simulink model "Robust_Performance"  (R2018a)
settings: Solver=ode113  StartTime=0.0  StopTime=20  FixedStep=0.0001  RelTol=1e-5  EnableMultiTasking=on
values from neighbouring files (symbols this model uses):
  d2r = pi/180    (= 0.0174532925199)    [init.m]
  Kr = Kq; Kr(3:4)=-Kq(3:4)    [init.m]
  Npv = 19    [init.m]    (also in Run_Robust_Performance.m; Run_Robustness.m)
  r2d = 1/d2r    (= 57.2957795131)    [init.m]
  Wf = 20    [init.m]
undefined symbols (not defined in the file or in its folder): Aa, Av, Ba, Bv, Ca, Cv, Da, Dv, Kq, TVC

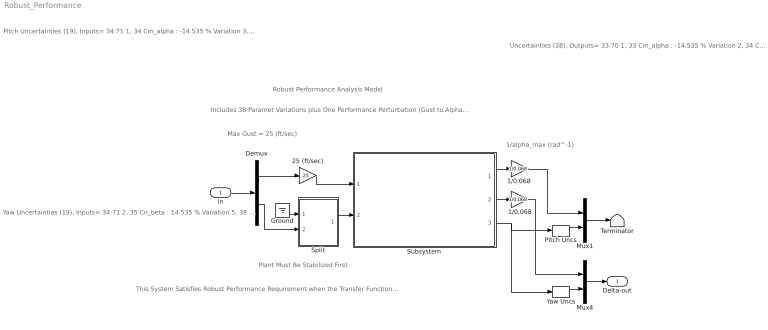
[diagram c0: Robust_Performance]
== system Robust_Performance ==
  note: Robust Performance Analysis Model
  note: Uncertainties (38), Outputs= 33:70 1, 33 Cm_alpha : -14.535 % Variation 2, 34 Cn_beta : 14.535 % Variation 3, 35 Ca_alpha : 17.153 % Variation 4, 36 Cz_alpha : -24.655 % Variation 5, 37 Cy_beta : -24.655 % Variation 6, 38 Cm_0 : -9.690 % Variation 7, 39 CZ_0 : -12.327 % Variation 8, 40 CA_0 : 6.679 % Variation 9, 41 I_xx : 19.786 % Variation 10, 42 I_yy : 14.153 % Variation 11, 43 I_zz : 14.158 % Variation 12, 44 Qbar : 9.865 % Variation 13, 45 Qbar : 9.865 % Variation 14, 46 Xcg locat: 3.492 % Variation 15, 47 Xcg locat: 3.492 % Variation 16, 48 Xcg locat: 3.492 % Variation 17, 49 M_slosh 1: 13.664 % Variation 18, 50 M_slosh 1: 13.664 % Variation 19, 51 X_slosh 1: 3.563 % Variation 20, 52 X_slosh 1: 3.563 % Variation 21, 53 X_slosh 1: 3.563 % Variation 22, 54 Wslsh_Y 1: 2.251 % Variation 23, 55 Wslsh_Z 1: 2.251 % Variation 24, 56 ZetSl_Y 1: 5.556 % Variation 25, 57 ZetSl_Z 1: 5.556 % Variation 26, 58 M_slosh 2: 14.465 % Variation 27, 59 M_slosh 2: 14.465 % Variation 28, 60 X_slosh 2: 7.956 % Variation 29, 61 X_slosh 2: 7.956 % Variation 30, 62 X_slosh 2: 7.956 % Variation 31, 63 Wslsh_Y 2: 2.251 % Variation 32, 64 Wslsh_Z 2: 2.251 % Variation 33, 65 ZetSl_Y 2: 6.667 % Variation 34, 66 ZetSl_Z 2: 6.667 % Variation 35, 67 W_flex 1: 5.000 Addit. Variat. 36, 68 W_flex 2: 5.000 Addit. Variat. 37, 69 W_flex 3: 8.000 Addit. Variat. 38, 70 W_flex 4: 8.000 Addit. Variat.
  note: Plant Must Be Stabilized First
  note: Includes 38 Paramet Variations plus One Performance Perturbation (Gust to Alpha or Beta)
  note: Pitch Uncertainties (19), Inputs= 34:71 1, 34 Cm_alpha : -14.535 % Variation 3, 36 Ca_alpha : 17.153 % Variation 4, 37 Cz_alpha : -24.655 % Variation 6, 39 Cm_0 : -9.690 % Variation 7, 40 CZ_0 : -12.327 % Variation 8, 41 CA_0 : 6.679 % Variation 10, 43 I_yy : 14.153 % Variation 12, 45 Qbar : 9.865 % Variation 15, 48 Xcg locat: 3.492 % Variation 18, 51 M_slosh 1: 13.664 % Variation 20, 53 X_slosh 1: 3.563 % Variation 23, 56 Wslsh_Z 1: 2.251 % Variation 25, 58 ZetSl_Z 1: 5.556 % Variation 27, 60 M_slosh 2: 14.465 % Variation 29, 62 X_slosh 2: 7.956 % Variation 32, 65 Wslsh_Z 2: 2.251 % Variation 34, 67 ZetSl_Z 2: 6.667 % Variation 36, 69 W_flex 2: 5.000 Addit. Variat. 38, 71 W_flex 4: 8.000 Addit. Variat.
  note: Yaw Uncertainties (19), Inputs= 34:71 2, 35 Cn_beta : 14.535 % Variation 5, 38 Cy_beta : -24.655 % Variation 9, 42 I_xx : 19.786 % Variation 11, 44 I_zz : 14.158 % Variation 13, 46 Qbar : 9.865 % Variation 14, 47 Xcg locat: 3.492 % Variation 16, 49 Xcg locat: 3.492 % Variation 17, 50 M_slosh 1: 13.664 % Variation 19, 52 X_slosh 1: 3.563 % Variation 21, 54 X_slosh 1: 3.563 % Variation 22, 55 Wslsh_Y 1: 2.251 % Variation 24, 57 ZetSl_Y 1: 5.556 % Variation 26, 59 M_slosh 2: 14.465 % Variation 28, 61 X_slosh 2: 7.956 % Variation 30, 63 X_slosh 2: 7.956 % Variation 31, 64 Wslsh_Y 2: 2.251 % Variation 33, 66 ZetSl_Y 2: 6.667 % Variation 35, 68 W_flex 1: 5.000 Addit. Variat. 37, 70 W_flex 3: 8.000 Addit. Variat.
  note: 1/alpha_max (rad^-1)
  note: Max Gust = 25 (ft/sec)
  note: This System Satisfies Robust Performance Requirement when the Transfer Function Magnitude is Less than One at All Frequencies. It Means that it will satisfy Both Performance to Gusts and its Stability will be Robust to All Parameter Variations Defined
  In : Inport
  1/0.068 : Gain  Gain=1/0.068
  "1/0.068 " : Gain  Gain=1/0.068
  25 (ft/sec) : Gain  Gain=25
  Demux : Demux  Outputs=[1, Npv]
  Ground : Ground
  Mux1 : Mux  Inputs=[1, Npv]
  Mux4 : Mux  Inputs=[1, Npv]
  Pitch Uncs : Selector  InputPortWidth=38  IndexOptions=Index vector (dialog)  Indices=[1,3,4,6,7,8,10,12,15,18,20,23,25,27,29,32,34,36,38]  OutputSizes=1
  Split : Subsystem
  Subsystem : Subsystem
  Terminator : Terminator
  Yaw Uncs : Selector  InputPortWidth=38  IndexOptions=Index vector (dialog)  Indices=[2,5,9,11,13,14,16,17,19,21,22,24,26,28,30,31,33,35,37]  OutputSizes=1
  Delta-out : Outport
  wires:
  Split/1(Delta-In) -> Subsystem/2(del-in)
  Subsystem/3(del-out) -> Yaw Uncs/1, Pitch Uncs/1
  Subsystem/2("beta ") -> 1/0.068/1
  Yaw Uncs/1 -> Mux4/2
  Subsystem/1(alpha) -> "1/0.068 "/1
  Pitch Uncs/1 -> Mux1/2
  In/1 -> Demux/1
  Demux/1 -> 25 (ft/sec)/1
  25 (ft/sec)/1 -> Subsystem/1(gust)
  "1/0.068 "/1 -> Mux1/1
  1/0.068/1 -> Mux4/1
  Ground/1 -> Split/1(Pitch)
  Demux/2 -> Split/2(Yaw)
  Mux4/1 -> Delta-out/1
  Mux1/1 -> Terminator/1

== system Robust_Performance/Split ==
  note: Pitch Uncertainties (19), Inputs= 34:71 1, 34 Cm_alpha : -14.535 % Variation 3, 36 Ca_alpha : 17.153 % Variation 4, 37 Cz_alpha : -24.655 % Variation 6, 39 Cm_0 : -9.690 % Variation 7, 40 CZ_0 : -12.327 % Variation 8, 41 CA_0 : 6.679 % Variation 10, 43 I_yy : 14.153 % Variation 12, 45 Qbar : 9.865 % Variation 15, 48 Xcg locat: 3.492 % Variation 18, 51 M_slosh 1: 13.664 % Variation 20, 53 X_slosh 1: 3.563 % Variation 23, 56 Wslsh_Z 1: 2.251 % Variation 25, 58 ZetSl_Z 1: 5.556 % Variation 27, 60 M_slosh 2: 14.465 % Variation 29, 62 X_slosh 2: 7.956 % Variation 32, 65 Wslsh_Z 2: 2.251 % Variation 34, 67 ZetSl_Z 2: 6.667 % Variation 36, 69 W_flex 2: 5.000 Addit. Variat. 38, 71 W_flex 4: 8.000 Addit. Variat.
  note: Uncertainties (38), Inputs= 34:71 1, 34 Cm_alpha : -14.535 % Variation 2, 35 Cn_beta : 14.535 % Variation 3, 36 Ca_alpha : 17.153 % Variation 4, 37 Cz_alpha : -24.655 % Variation 5, 38 Cy_beta : -24.655 % Variation 6, 39 Cm_0 : -9.690 % Variation 7, 40 CZ_0 : -12.327 % Variation 8, 41 CA_0 : 6.679 % Variation 9, 42 I_xx : 19.786 % Variation 10, 43 I_yy : 14.153 % Variation 11, 44 I_zz : 14.158 % Variation 12, 45 Qbar : 9.865 % Variation 13, 46 Qbar : 9.865 % Variation 14, 47 Xcg locat: 3.492 % Variation 15, 48 Xcg locat: 3.492 % Variation 16, 49 Xcg locat: 3.492 % Variation 17, 50 M_slosh 1: 13.664 % Variation 18, 51 M_slosh 1: 13.664 % Variation 19, 52 X_slosh 1: 3.563 % Variation 20, 53 X_slosh 1: 3.563 % Variation 21, 54 X_slosh 1: 3.563 % Variation 22, 55 Wslsh_Y 1: 2.251 % Variation 23, 56 Wslsh_Z 1: 2.251 % Variation 24, 57 ZetSl_Y 1: 5.556 % Variation 25, 58 ZetSl_Z 1: 5.556 % Variation 26, 59 M_slosh 2: 14.465 % Variation 27, 60 M_slosh 2: 14.465 % Variation 28, 61 X_slosh 2: 7.956 % Variation 29, 62 X_slosh 2: 7.956 % Variation 30, 63 X_slosh 2: 7.956 % Variation 31, 64 Wslsh_Y 2: 2.251 % Variation 32, 65 Wslsh_Z 2: 2.251 % Variation 33, 66 ZetSl_Y 2: 6.667 % Variation 34, 67 ZetSl_Z 2: 6.667 % Variation 35, 68 W_flex 1: 5.000 Addit. Variat. 36, 69 W_flex 2: 5.000 Addit. Variat. 37, 70 W_flex 3: 8.000 Addit. Variat. 38, 71 W_flex 4: 8.000 Addit. Variat.
  note: Yaw Uncertainties (19), Inputs= 34:71 2, 35 Cn_beta : 14.535 % Variation 5, 38 Cy_beta : -24.655 % Variation 9, 42 I_xx : 19.786 % Variation 11, 44 I_zz : 14.158 % Variation 13, 46 Qbar : 9.865 % Variation 14, 47 Xcg locat: 3.492 % Variation 16, 49 Xcg locat: 3.492 % Variation 17, 50 M_slosh 1: 13.664 % Variation 19, 52 X_slosh 1: 3.563 % Variation 21, 54 X_slosh 1: 3.563 % Variation 22, 55 Wslsh_Y 1: 2.251 % Variation 24, 57 ZetSl_Y 1: 5.556 % Variation 26, 59 M_slosh 2: 14.465 % Variation 28, 61 X_slosh 2: 7.956 % Variation 30, 63 X_slosh 2: 7.956 % Variation 31, 64 Wslsh_Y 2: 2.251 % Variation 33, 66 ZetSl_Y 2: 6.667 % Variation 35, 68 W_flex 1: 5.000 Addit. Variat. 37, 70 W_flex 3: 8.000 Addit. Variat.
  Pitch : Inport
  Yaw : Inport  Port=2
  Demux : Demux  Outputs=19
  Demux1 : Demux  Outputs=19
  Mux : Mux  Inputs=38
  Delta-In : Outport
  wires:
  Pitch/1 -> Demux/1
  Demux/1 -> Mux/1
  Demux/2 -> Mux/3
  Demux/4 -> Mux/6
  Demux/3 -> Mux/4
  Demux/5 -> Mux/7
  Demux/6 -> Mux/8
  Demux/7 -> Mux/10
  Demux/8 -> Mux/12
  Demux/9 -> Mux/15
  Demux/10 -> Mux/18
  Demux/11 -> Mux/20
  Demux/12 -> Mux/23
  Demux/13 -> Mux/25
  Demux/14 -> Mux/27
  Demux/15 -> Mux/29
  Demux/16 -> Mux/32
  Demux/17 -> Mux/34
  Demux/18 -> Mux/36
  Demux/19 -> Mux/38
  Yaw/1 -> Demux1/1
  Demux1/19 -> Mux/37
  Demux1/18 -> Mux/35
  Demux1/17 -> Mux/33
  Demux1/16 -> Mux/31
  Demux1/15 -> Mux/30
  Demux1/14 -> Mux/28
  Demux1/13 -> Mux/26
  Demux1/12 -> Mux/24
  Demux1/11 -> Mux/22
  Demux1/10 -> Mux/21
  Demux1/9 -> Mux/19
  Demux1/8 -> Mux/17
  Demux1/7 -> Mux/16
  Demux1/1 -> Mux/2
  Demux1/2 -> Mux/5
  Demux1/3 -> Mux/9
  Demux1/4 -> Mux/11
  Demux1/5 -> Mux/13
  Demux1/6 -> Mux/14
  Mux/1 -> Delta-In/1

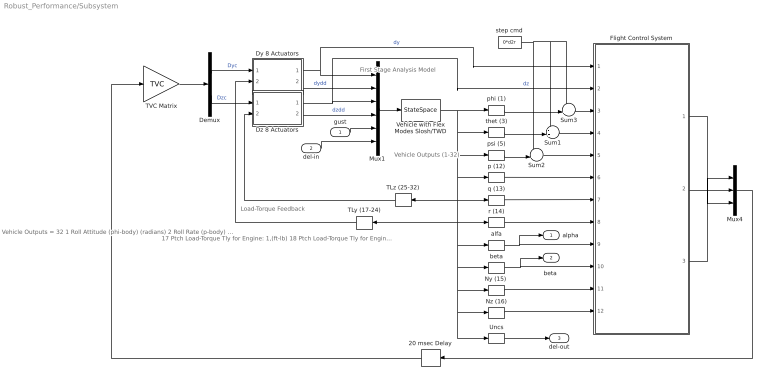
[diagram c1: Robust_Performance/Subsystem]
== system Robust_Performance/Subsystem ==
  note: First Stage Analysis Model
  note: Load-Torque Feedback
  note: 17 Ptch Load-Torque Tly for Engine: 1,(ft-lb) 18 Ptch Load-Torque Tly for Engine: 2,(ft-lb) 19 Ptch Load-Torque Tly for Engine: 3,(ft-lb) 20 Ptch Load-Torque Tly for Engine: 4,(ft-lb) 21 Ptch Load-Torque Tly for Engine: 5,(ft-lb) 22 Ptch Load-Torque Tly for Engine: 6,(ft-lb) 23 Ptch Load-Torque Tly for Engine: 7,(ft-lb) 24 Ptch Load-Torque Tly for Engine: 8,(ft-lb) 25 Yaw Load-Torque Tlz for Engine: 1,(ft-lb) 26 Yaw Load-Torque Tlz for Engine: 2,(ft-lb) 27 Yaw Load-Torque Tlz for Engine: 3,(ft-lb) 28 Yaw Load-Torque Tlz for Engine: 4,(ft-lb) 29 Yaw Load-Torque Tlz for Engine: 5,(ft-lb) 30 Yaw Load-Torque Tlz for Engine: 6,(ft-lb) 31 Yaw Load-Torque Tlz for Engine: 7,(ft-lb) 32 Yaw Load-Torque Tlz for Engine: 8,(ft-lb)
  note: Vehicle Outputs = 32 1 Roll Attitude (phi-body) (radians) 2 Roll Rate (p-body) (rad/sec) 3 Pitch Attitude (thet-bdy) (radians) 4 Pitch Rate (q-body) (rad/sec) 5 Yaw Attitude (psi-body) (radians) 6 Yaw Rate (r-body) (rad/sec) 7 Angle of attack, alfa, (radians) 8 Angle of sideslip, beta, (radian) 9 Change in Altitude, delta-h, (feet) 10 Forward Acceleration (V-dot) (ft/sec) 11 Cross Range Velocity (Vcr) (ft/sec) 12 Rate-Gyro # 1, Roll Rate (Body) (rad/sec) 13 Rate-Gyro # 2, Pitch Rate (Body) (rad/sec) 14 Rate-Gyro # 3, Yaw Rate (Body) (rad/sec) 15 Accelerom # 1, (along Y), (ft/sec^2) Translat. Accelerat. 16 Accelerom # 2, (along Z), (ft/sec^2) Translat. Accelerat.
  note: Vehicle Outputs (1-32)
  gust : Inport
  del-in : Inport  Port=2
  20 msec Delay : TransportDelay  DelayTime="[1  1  1]*0.02"  InitialOutput="[0  0  0]"  PadeOrder=2
  Demux : Demux  Outputs=[8, 8]
  Dy 8 Actuators : Subsystem
  Dz 8 Actuators : Subsystem
  Flight Control System : Subsystem
  Mux1 : Mux  Inputs=[8, 8, 8, 8, 1, 38]
  Mux4 : Mux  Inputs=3
  "Ny (15) " : Selector  InputPortWidth=70  IndexOptions=Index vector (dialog)  Indices=[15]  OutputSizes=1
  Nz (16) : Selector  InputPortWidth=70  IndexOptions=Index vector (dialog)  Indices=[16]  OutputSizes=1
  Sum1 : Sum  Inputs=-+|
  Sum2 : Sum  Inputs=-+|
  Sum3 : Sum  Inputs=-+|
  TLy (17-24) : Selector  InputPortWidth=70  IndexOptions=Index vector (dialog)  Indices=[17:24]  OutputSizes=1
  TLz (25-32) : Selector  InputPortWidth=70  IndexOptions=Index vector (dialog)  Indices=[25:32]  OutputSizes=1
  TVC Matrix : Gain  Gain=TVC  Multiplication=Matrix(K*u)
  Uncs : Selector  InputPortWidth=70  IndexOptions=Index vector (dialog)  Indices=[33:70]  OutputSizes=1
  Vehicle with Flex Modes Slosh/TWD : StateSpace  A=Av  B=Bv  C=Cv  D=Dv  InitialCondition=0
  alfa : Selector  InputPortWidth=70  IndexOptions=Index vector (dialog)  Indices=[7]  OutputSizes=1
  beta : Selector  InputPortWidth=70  IndexOptions=Index vector (dialog)  Indices=[8]  OutputSizes=1
  p (12) : Selector  InputPortWidth=70  IndexOptions=Index vector (dialog)  Indices=[12]  OutputSizes=1
  phi (1) : Selector  InputPortWidth=70  IndexOptions=Index vector (dialog)  Indices=[1]  OutputSizes=1
  psi (5) : Selector  InputPortWidth=70  IndexOptions=Index vector (dialog)  Indices=[5]  OutputSizes=1
  q (13) : Selector  InputPortWidth=70  IndexOptions=Index vector (dialog)  Indices=[13]  OutputSizes=1
  r (14) : Selector  InputPortWidth=70  IndexOptions=Index vector (dialog)  Indices=[14]  OutputSizes=1
  step cmd : Constant  Value=0*d2r
  thet (3) : Selector  InputPortWidth=70  IndexOptions=Index vector (dialog)  Indices=[3]  OutputSizes=1
  alpha : Outport
  "beta " : Outport  Port=2
  del-out : Outport  Port=3
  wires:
  Mux1/1 -> Vehicle with Flex Modes Slosh/TWD/1
  Dz 8 Actuators/2(dzdd) -> Mux1/4  "dzdd"
  p (12)/1 -> Flight Control System/6(p)
  Vehicle with Flex Modes Slosh/TWD/1 -> TLz (25-32)/1, "Ny (15) "/1, Uncs/1, Nz (16)/1, beta/1, alfa/1, TLy (17-24)/1, r (14)/1, q (13)/1, p (12)/1, psi (5)/1, thet (3)/1, phi (1)/1
  20 msec Delay/1 -> TVC Matrix/1
  TVC Matrix/1 -> Demux/1
  gust/1 -> Mux1/5
  del-in/1 -> Mux1/6
  "Ny (15) "/1 -> Flight Control System/11(NY)
  Dz 8 Actuators/1(dz) -> Flight Control System/2(dz), Mux1/3  "dz"
  r (14)/1 -> Flight Control System/8(r)
  step cmd/1 -> Sum1/1, Sum3/1, Sum2/1
  TLy (17-24)/1 -> Dy 8 Actuators/2(TLy)
  TLz (25-32)/1 -> Dz 8 Actuators/2(TLz)
  alfa/1 -> Flight Control System/9(alfa), alpha/1
  Flight Control System/2(DQ_tvc) -> Mux4/2
  Flight Control System/1(DP_tvc) -> Mux4/1
  Dy 8 Actuators/1(dy) -> Flight Control System/1(dy), Mux1/1  "dy"
  q (13)/1 -> Flight Control System/7(q)
  Dy 8 Actuators/2(dydd) -> Mux1/2  "dydd"
  beta/1 -> Flight Control System/10(beta), "beta "/1
  Flight Control System/3(DR_tvc) -> Mux4/3
  psi (5)/1 -> Sum2/2
  Demux/2 -> Dz 8 Actuators/1(dzc)  "Dzc"
  Sum2/1 -> Flight Control System/5(psi)
  Sum3/1 -> Flight Control System/3(phi)
  Sum1/1 -> Flight Control System/4(thet)
  Nz (16)/1 -> Flight Control System/12(NZ)
  thet (3)/1 -> Sum1/2
  Demux/1 -> Dy 8 Actuators/1(dyc)  "Dyc"
  phi (1)/1 -> Sum3/2
  Mux4/1 -> 20 msec Delay/1
  Uncs/1 -> del-out/1

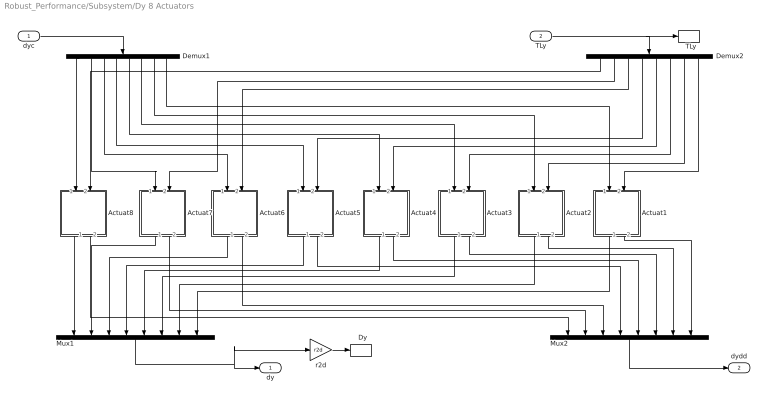
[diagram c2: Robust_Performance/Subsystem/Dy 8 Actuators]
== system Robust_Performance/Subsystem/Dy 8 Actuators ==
  dyc : Inport
  TLy : Inport  Port=2
  "  Dy" : ToWorkspace  VariableName=DY  SampleTime=-1
  "  TLy" : ToWorkspace  VariableName=TLy  SampleTime=-1
  Actuat1 : Subsystem
  Actuat2 : Subsystem
  Actuat3 : Subsystem
  Actuat4 : Subsystem
  Actuat5 : Subsystem
  Actuat6 : Subsystem
  Actuat7 : Subsystem
  Actuat8 : Subsystem
  Demux1 : Demux  Outputs=8
  Demux2 : Demux  Outputs=8
  Mux1 : Mux  Inputs=8
  Mux2 : Mux  Inputs=8
  r2d : Gain  Gain=r2d
  dy : Outport
  dydd : Outport  Port=2
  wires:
  TLy/1 -> "  TLy"/1, Demux2/1
  Mux2/1 -> dydd/1
  Actuat5/1(dout) -> Mux1/4
  Demux1/5 -> Actuat4/1(delin)
  Actuat3/2(ddot) -> Mux2/6
  Actuat8/1(dout) -> Mux1/1
  Demux1/4 -> Actuat5/1(delin)
  Actuat1/1(dout) -> Mux1/8
  Actuat4/2(ddot) -> Mux2/5
  Actuat4/1(dout) -> Mux1/5
  Demux2/4 -> Actuat5/2(TL)
  Demux2/6 -> Actuat3/2(TL)
  Demux2/7 -> Actuat2/2(TL)
  Actuat6/2(ddot) -> Mux2/3
  Demux2/2 -> Actuat7/2(TL)
  Actuat5/2(ddot) -> Mux2/4
  Demux1/3 -> Actuat6/1(delin)
  Actuat2/2(ddot) -> Mux2/7
  Actuat8/2(ddot) -> Mux2/1
  dyc/1 -> Demux1/1
  Mux1/1 -> r2d/1, dy/1
  Actuat1/2(ddot) -> Mux2/8
  Actuat7/2(ddot) -> Mux2/2
  Demux1/2 -> Actuat7/1(delin)
  Demux1/7 -> Actuat2/1(delin)
  Demux1/8 -> Actuat1/1(delin)
  Actuat7/1(dout) -> Mux1/2
  Demux2/5 -> Actuat4/2(TL)
  Demux1/1 -> Actuat8/1(delin)
  Demux2/1 -> Actuat8/2(TL)
  Actuat2/1(dout) -> Mux1/7
  Demux2/8 -> Actuat1/2(TL)
  Demux2/3 -> Actuat6/2(TL)
  Actuat3/1(dout) -> Mux1/6
  Actuat6/1(dout) -> Mux1/3
  Demux1/6 -> Actuat3/1(delin)
  r2d/1 -> "  Dy"/1

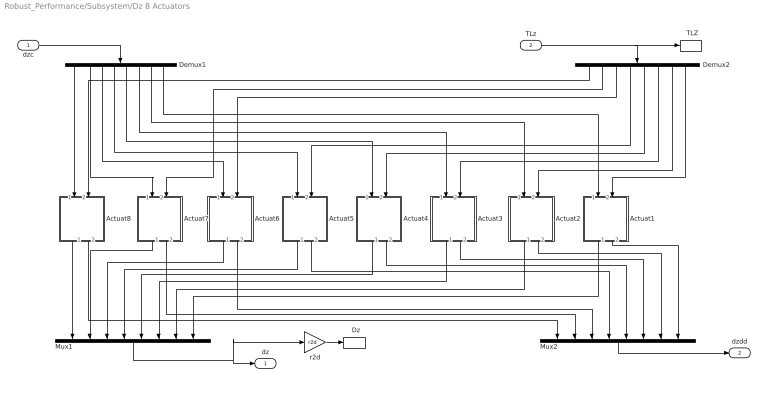
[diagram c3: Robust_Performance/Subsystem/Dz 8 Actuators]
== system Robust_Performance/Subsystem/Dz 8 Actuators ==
  dzc : Inport
  TLz : Inport  Port=2
  "  Dz" : ToWorkspace  VariableName=DZ  SampleTime=-1
  "  TLZ" : ToWorkspace  VariableName=TLz  SampleTime=-1
  Actuat1 : Subsystem
  Actuat2 : Subsystem
  Actuat3 : Subsystem
  Actuat4 : Subsystem
  Actuat5 : Subsystem
  Actuat6 : Subsystem
  Actuat7 : Subsystem
  Actuat8 : Subsystem
  Demux1 : Demux  Outputs=8
  Demux2 : Demux  Outputs=8
  Mux1 : Mux  Inputs=8
  Mux2 : Mux  Inputs=8
  r2d : Gain  Gain=r2d
  dz : Outport
  dzdd : Outport  Port=2
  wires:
  TLz/1 -> "  TLZ"/1, Demux2/1
  Mux2/1 -> dzdd/1
  Actuat5/1(dout) -> Mux1/4
  Demux1/5 -> Actuat4/1(delin)
  Actuat3/2(ddot) -> Mux2/6
  Actuat8/1(dout) -> Mux1/1
  Demux1/4 -> Actuat5/1(delin)
  Actuat1/1(dout) -> Mux1/8
  Actuat4/2(ddot) -> Mux2/5
  Actuat4/1(dout) -> Mux1/5
  Demux2/4 -> Actuat5/2(TL)
  Demux2/6 -> Actuat3/2(TL)
  Demux2/7 -> Actuat2/2(TL)
  Actuat6/2(ddot) -> Mux2/3
  Demux2/2 -> Actuat7/2(TL)
  Actuat5/2(ddot) -> Mux2/4
  Demux1/3 -> Actuat6/1(delin)
  Actuat2/2(ddot) -> Mux2/7
  Actuat8/2(ddot) -> Mux2/1
  dzc/1 -> Demux1/1
  Mux1/1 -> r2d/1, dz/1
  Actuat1/2(ddot) -> Mux2/8
  Actuat7/2(ddot) -> Mux2/2
  Demux1/2 -> Actuat7/1(delin)
  Demux1/7 -> Actuat2/1(delin)
  Demux1/8 -> Actuat1/1(delin)
  Actuat7/1(dout) -> Mux1/2
  Demux2/5 -> Actuat4/2(TL)
  Demux1/1 -> Actuat8/1(delin)
  Demux2/1 -> Actuat8/2(TL)
  Actuat2/1(dout) -> Mux1/7
  Demux2/8 -> Actuat1/2(TL)
  Demux2/3 -> Actuat6/2(TL)
  Actuat3/1(dout) -> Mux1/6
  Actuat6/1(dout) -> Mux1/3
  Demux1/6 -> Actuat3/1(delin)
  r2d/1 -> "  Dz"/1

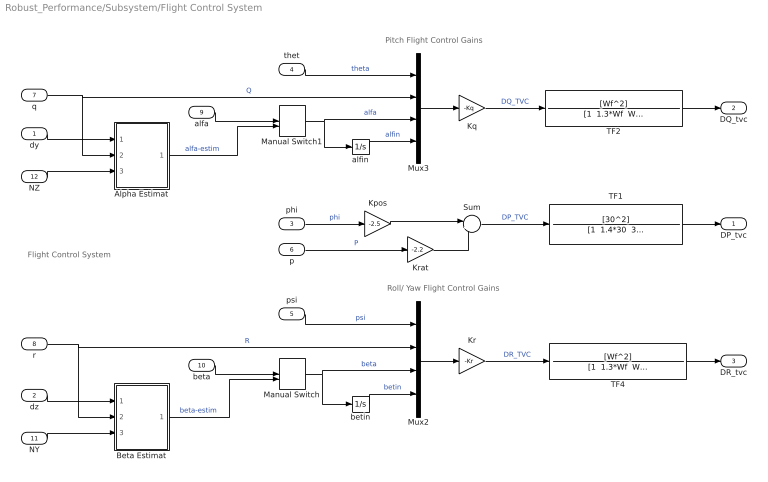
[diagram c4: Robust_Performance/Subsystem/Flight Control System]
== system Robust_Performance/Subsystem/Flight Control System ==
  note: Pitch Flight Control Gains
  note: Roll/ Yaw Flight Control Gains
  note: Flight Control System
  dy : Inport
  dz : Inport  Port=2
  phi : Inport  Port=3
  thet : Inport  Port=4
  psi : Inport  Port=5
  p : Inport  Port=6
  q : Inport  Port=7
  r : Inport  Port=8
  alfa : Inport  Port=9
  beta : Inport  Port=10
  NY : Inport  Port=11
  NZ : Inport  Port=12
  Alpha Estimat : Subsystem
  Beta Estimat : Subsystem
  Kpos : Gain  Gain=-2.5  Multiplication=Matrix(K*u)
  Kq : Gain  Gain=-Kq  Multiplication=Matrix(K*u)
  Kr : Gain  Gain=-Kr  Multiplication=Matrix(K*u)
  Krat : Gain  Gain=-2.2  Multiplication=Matrix(K*u)
  Manual Switch : ManualSwitch  CurrentSetting=0
  Manual Switch1 : ManualSwitch  CurrentSetting=0
  Mux2 : Mux
  Mux3 : Mux
  Sum : Sum  Inputs=|++
  TF1 : TransferFcn  Numerator=[30^2]  Denominator="[1  1.4*30  30^2]"
  TF2 : TransferFcn  Numerator=[Wf^2]  Denominator="[1  1.3*Wf  Wf^2]"
  TF4 : TransferFcn  Numerator=[Wf^2]  Denominator="[1  1.3*Wf  Wf^2]"
  alfin : Integrator
  betin : Integrator
  DP_tvc : Outport
  DQ_tvc : Outport  Port=2
  DR_tvc : Outport  Port=3
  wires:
  Alpha Estimat/1(alfest) -> Manual Switch1/2  "alfa-estim"
  alfa/1 -> Manual Switch1/1
  Manual Switch1/1 -> Mux3/3, alfin/1  "alfa"
  beta/1 -> Manual Switch/1
  Manual Switch/1 -> betin/1, Mux2/3  "beta"
  psi/1 -> Mux2/1  "psi"
  betin/1 -> Mux2/4  "betin"
  q/1 -> Alpha Estimat/2(q), Mux3/2  "Q"
  r/1 -> Mux2/2, Beta Estimat/2(r)  "R"
  alfin/1 -> Mux3/4  "alfin"
  thet/1 -> Mux3/1  "theta"
  Kq/1 -> TF2/1  "DQ_TVC"
  NZ/1 -> Alpha Estimat/3(Zdd)
  NY/1 -> Beta Estimat/3(Ydd)
  Beta Estimat/1(betest) -> Manual Switch/2  "beta-estim"
  dy/1 -> Alpha Estimat/1(dy)
  dz/1 -> Beta Estimat/1(dz)
  Mux3/1 -> Kq/1
  Kpos/1 -> Sum/1
  Sum/1 -> TF1/1  "DP_TVC"
  Krat/1 -> Sum/2
  p/1 -> Krat/1  "P"
  phi/1 -> Kpos/1  "phi"
  Mux2/1 -> Kr/1
  TF1/1 -> DP_tvc/1
  TF2/1 -> DQ_tvc/1
  Kr/1 -> TF4/1  "DR_TVC"
  TF4/1 -> DR_tvc/1

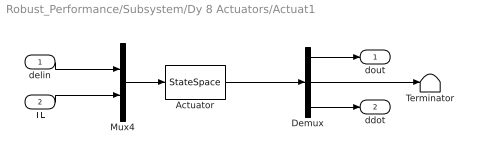
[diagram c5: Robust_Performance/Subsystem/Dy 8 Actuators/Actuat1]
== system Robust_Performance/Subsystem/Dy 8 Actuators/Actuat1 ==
  delin : Inport
  TL : Inport  Port=2
  Actuator : StateSpace  A=Aa  B=Ba  C=Ca  D=Da  InitialCondition=0
  Demux : Demux  Outputs=3
  Mux4 : Mux  Inputs=2
  Terminator : Terminator
  dout : Outport
  ddot : Outport  Port=2
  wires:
  Demux/3 -> ddot/1
  TL/1 -> Mux4/2
  Mux4/1 -> Actuator/1
  Actuator/1 -> Demux/1
  delin/1 -> Mux4/1
  Demux/1 -> dout/1
  Demux/2 -> Terminator/1

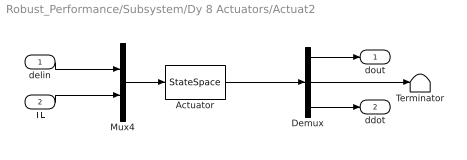
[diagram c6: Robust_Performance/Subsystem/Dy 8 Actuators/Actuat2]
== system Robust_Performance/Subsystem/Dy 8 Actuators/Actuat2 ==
  delin : Inport
  TL : Inport  Port=2
  Actuator : StateSpace  A=Aa  B=Ba  C=Ca  D=Da  InitialCondition=0
  Demux : Demux  Outputs=3
  Mux4 : Mux  Inputs=2
  Terminator : Terminator
  dout : Outport
  ddot : Outport  Port=2
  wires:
  Demux/3 -> ddot/1
  TL/1 -> Mux4/2
  Mux4/1 -> Actuator/1
  Actuator/1 -> Demux/1
  delin/1 -> Mux4/1
  Demux/1 -> dout/1
  Demux/2 -> Terminator/1

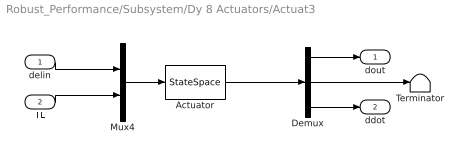
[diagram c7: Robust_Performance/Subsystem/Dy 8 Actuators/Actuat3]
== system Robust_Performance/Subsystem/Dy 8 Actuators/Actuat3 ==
  delin : Inport
  TL : Inport  Port=2
  Actuator : StateSpace  A=Aa  B=Ba  C=Ca  D=Da  InitialCondition=0
  Demux : Demux  Outputs=3
  Mux4 : Mux  Inputs=2
  Terminator : Terminator
  dout : Outport
  ddot : Outport  Port=2
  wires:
  Demux/3 -> ddot/1
  TL/1 -> Mux4/2
  Mux4/1 -> Actuator/1
  Actuator/1 -> Demux/1
  delin/1 -> Mux4/1
  Demux/1 -> dout/1
  Demux/2 -> Terminator/1

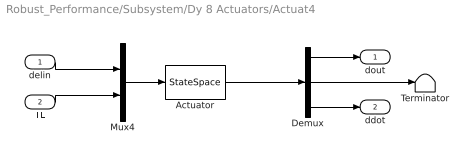
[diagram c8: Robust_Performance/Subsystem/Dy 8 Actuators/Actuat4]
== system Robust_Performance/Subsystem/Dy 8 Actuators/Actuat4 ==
  delin : Inport
  TL : Inport  Port=2
  Actuator : StateSpace  A=Aa  B=Ba  C=Ca  D=Da  InitialCondition=0
  Demux : Demux  Outputs=3
  Mux4 : Mux  Inputs=2
  Terminator : Terminator
  dout : Outport
  ddot : Outport  Port=2
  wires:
  Demux/3 -> ddot/1
  TL/1 -> Mux4/2
  Mux4/1 -> Actuator/1
  Actuator/1 -> Demux/1
  delin/1 -> Mux4/1
  Demux/1 -> dout/1
  Demux/2 -> Terminator/1

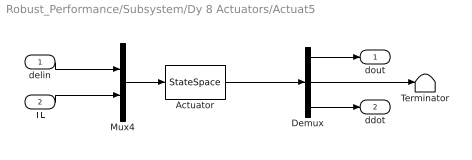
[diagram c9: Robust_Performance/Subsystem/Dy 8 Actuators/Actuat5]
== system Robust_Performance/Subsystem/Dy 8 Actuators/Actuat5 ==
  delin : Inport
  TL : Inport  Port=2
  Actuator : StateSpace  A=Aa  B=Ba  C=Ca  D=Da  InitialCondition=0
  Demux : Demux  Outputs=3
  Mux4 : Mux  Inputs=2
  Terminator : Terminator
  dout : Outport
  ddot : Outport  Port=2
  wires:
  Demux/3 -> ddot/1
  TL/1 -> Mux4/2
  Mux4/1 -> Actuator/1
  Actuator/1 -> Demux/1
  delin/1 -> Mux4/1
  Demux/1 -> dout/1
  Demux/2 -> Terminator/1

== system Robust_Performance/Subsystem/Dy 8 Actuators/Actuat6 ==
  delin : Inport
  TL : Inport  Port=2
  Actuator : StateSpace  A=Aa  B=Ba  C=Ca  D=Da  InitialCondition=0
  Demux : Demux  Outputs=3
  Mux4 : Mux  Inputs=2
  Terminator : Terminator
  dout : Outport
  ddot : Outport  Port=2
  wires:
  Demux/3 -> ddot/1
  TL/1 -> Mux4/2
  Mux4/1 -> Actuator/1
  Actuator/1 -> Demux/1
  delin/1 -> Mux4/1
  Demux/1 -> dout/1
  Demux/2 -> Terminator/1

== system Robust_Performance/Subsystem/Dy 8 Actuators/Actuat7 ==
  delin : Inport
  TL : Inport  Port=2
  Actuator : StateSpace  A=Aa  B=Ba  C=Ca  D=Da  InitialCondition=0
  Demux : Demux  Outputs=3
  Mux4 : Mux  Inputs=2
  Terminator : Terminator
  dout : Outport
  ddot : Outport  Port=2
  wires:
  Demux/3 -> ddot/1
  TL/1 -> Mux4/2
  Mux4/1 -> Actuator/1
  Actuator/1 -> Demux/1
  delin/1 -> Mux4/1
  Demux/1 -> dout/1
  Demux/2 -> Terminator/1

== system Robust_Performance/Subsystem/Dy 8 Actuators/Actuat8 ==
  delin : Inport
  TL : Inport  Port=2
  Actuator : StateSpace  A=Aa  B=Ba  C=Ca  D=Da  InitialCondition=0
  Demux : Demux  Outputs=3
  Mux4 : Mux  Inputs=2
  Terminator : Terminator
  dout : Outport
  ddot : Outport  Port=2
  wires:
  Demux/3 -> ddot/1
  TL/1 -> Mux4/2
  Mux4/1 -> Actuator/1
  Actuator/1 -> Demux/1
  delin/1 -> Mux4/1
  Demux/1 -> dout/1
  Demux/2 -> Terminator/1

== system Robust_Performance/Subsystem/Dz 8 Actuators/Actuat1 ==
  delin : Inport
  TL : Inport  Port=2
  Actuator : StateSpace  A=Aa  B=Ba  C=Ca  D=Da  InitialCondition=0
  Demux : Demux  Outputs=3
  Mux4 : Mux  Inputs=2
  Terminator : Terminator
  dout : Outport
  ddot : Outport  Port=2
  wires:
  Demux/3 -> ddot/1
  TL/1 -> Mux4/2
  Mux4/1 -> Actuator/1
  Actuator/1 -> Demux/1
  delin/1 -> Mux4/1
  Demux/1 -> dout/1
  Demux/2 -> Terminator/1

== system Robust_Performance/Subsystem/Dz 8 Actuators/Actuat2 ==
  delin : Inport
  TL : Inport  Port=2
  Actuator : StateSpace  A=Aa  B=Ba  C=Ca  D=Da  InitialCondition=0
  Demux : Demux  Outputs=3
  Mux4 : Mux  Inputs=2
  Terminator : Terminator
  dout : Outport
  ddot : Outport  Port=2
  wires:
  Demux/3 -> ddot/1
  TL/1 -> Mux4/2
  Mux4/1 -> Actuator/1
  Actuator/1 -> Demux/1
  delin/1 -> Mux4/1
  Demux/1 -> dout/1
  Demux/2 -> Terminator/1

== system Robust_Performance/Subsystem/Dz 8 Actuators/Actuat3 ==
  delin : Inport
  TL : Inport  Port=2
  Actuator : StateSpace  A=Aa  B=Ba  C=Ca  D=Da  InitialCondition=0
  Demux : Demux  Outputs=3
  Mux4 : Mux  Inputs=2
  Terminator : Terminator
  dout : Outport
  ddot : Outport  Port=2
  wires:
  Demux/3 -> ddot/1
  TL/1 -> Mux4/2
  Mux4/1 -> Actuator/1
  Actuator/1 -> Demux/1
  delin/1 -> Mux4/1
  Demux/1 -> dout/1
  Demux/2 -> Terminator/1

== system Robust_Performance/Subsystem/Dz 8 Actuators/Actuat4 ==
  delin : Inport
  TL : Inport  Port=2
  Actuator : StateSpace  A=Aa  B=Ba  C=Ca  D=Da  InitialCondition=0
  Demux : Demux  Outputs=3
  Mux4 : Mux  Inputs=2
  Terminator : Terminator
  dout : Outport
  ddot : Outport  Port=2
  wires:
  Demux/3 -> ddot/1
  TL/1 -> Mux4/2
  Mux4/1 -> Actuator/1
  Actuator/1 -> Demux/1
  delin/1 -> Mux4/1
  Demux/1 -> dout/1
  Demux/2 -> Terminator/1

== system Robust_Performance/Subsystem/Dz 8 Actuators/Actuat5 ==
  delin : Inport
  TL : Inport  Port=2
  Actuator : StateSpace  A=Aa  B=Ba  C=Ca  D=Da  InitialCondition=0
  Demux : Demux  Outputs=3
  Mux4 : Mux  Inputs=2
  Terminator : Terminator
  dout : Outport
  ddot : Outport  Port=2
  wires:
  Demux/3 -> ddot/1
  TL/1 -> Mux4/2
  Mux4/1 -> Actuator/1
  Actuator/1 -> Demux/1
  delin/1 -> Mux4/1
  Demux/1 -> dout/1
  Demux/2 -> Terminator/1

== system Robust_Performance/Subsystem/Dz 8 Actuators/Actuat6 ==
  delin : Inport
  TL : Inport  Port=2
  Actuator : StateSpace  A=Aa  B=Ba  C=Ca  D=Da  InitialCondition=0
  Demux : Demux  Outputs=3
  Mux4 : Mux  Inputs=2
  Terminator : Terminator
  dout : Outport
  ddot : Outport  Port=2
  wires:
  Demux/3 -> ddot/1
  TL/1 -> Mux4/2
  Mux4/1 -> Actuator/1
  Actuator/1 -> Demux/1
  delin/1 -> Mux4/1
  Demux/1 -> dout/1
  Demux/2 -> Terminator/1

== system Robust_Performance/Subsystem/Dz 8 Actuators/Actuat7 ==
  delin : Inport
  TL : Inport  Port=2
  Actuator : StateSpace  A=Aa  B=Ba  C=Ca  D=Da  InitialCondition=0
  Demux : Demux  Outputs=3
  Mux4 : Mux  Inputs=2
  Terminator : Terminator
  dout : Outport
  ddot : Outport  Port=2
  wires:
  Demux/3 -> ddot/1
  TL/1 -> Mux4/2
  Mux4/1 -> Actuator/1
  Actuator/1 -> Demux/1
  delin/1 -> Mux4/1
  Demux/1 -> dout/1
  Demux/2 -> Terminator/1

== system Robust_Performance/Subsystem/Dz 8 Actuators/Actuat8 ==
  delin : Inport
  TL : Inport  Port=2
  Actuator : StateSpace  A=Aa  B=Ba  C=Ca  D=Da  InitialCondition=0
  Demux : Demux  Outputs=3
  Mux4 : Mux  Inputs=2
  Terminator : Terminator
  dout : Outport
  ddot : Outport  Port=2
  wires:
  Demux/3 -> ddot/1
  TL/1 -> Mux4/2
  Mux4/1 -> Actuator/1
  Actuator/1 -> Demux/1
  delin/1 -> Mux4/1
  Demux/1 -> dout/1
  Demux/2 -> Terminator/1

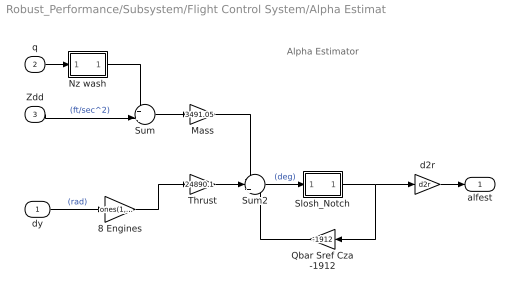
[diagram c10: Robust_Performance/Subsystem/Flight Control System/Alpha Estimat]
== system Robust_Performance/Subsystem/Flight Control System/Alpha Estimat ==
  note: Alpha Estimator
  dy : Inport
  q : Inport  Port=2
  Zdd : Inport  Port=3
  8 Engines : Gain  Gain=ones(1,8)  Multiplication=Matrix(K*u) (u vector)
  Mass : Gain  Gain=3491.05
  Nz wash : Subsystem
  Qbar Sref Cza -1912 : Gain  Gain=-1912
  Slosh_Notch : Subsystem
  Sum : Sum  Inputs=++|
  Sum2 : Sum  Inputs=--+
  Thrust : Gain  Gain=24890.1
  d2r : Gain  Gain=d2r
  alfest : Outport
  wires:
  dy/1 -> 8 Engines/1  "(rad)"
  Sum/1 -> Mass/1
  q/1 -> Nz wash/1(in)
  d2r/1 -> alfest/1
  Zdd/1 -> Sum/2  "(ft/sec^2)"
  Qbar Sref Cza -1912/1 -> Sum2/3
  Sum2/1 -> Slosh_Notch/1(in)  "(deg)"
  Nz wash/1(ou) -> Sum/1
  Slosh_Notch/1(ou) -> d2r/1, Qbar Sref Cza -1912/1
  Mass/1 -> Sum2/1
  Thrust/1 -> Sum2/2
  8 Engines/1 -> Thrust/1

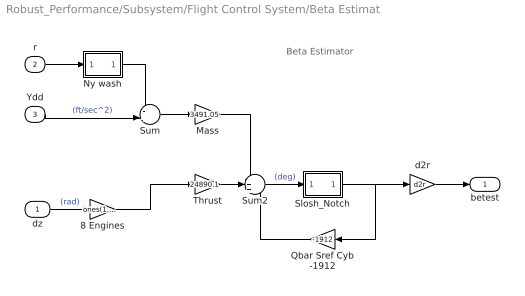
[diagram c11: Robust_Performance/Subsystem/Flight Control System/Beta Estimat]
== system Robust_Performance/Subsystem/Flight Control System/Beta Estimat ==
  note: Beta Estimator
  dz : Inport
  r : Inport  Port=2
  Ydd : Inport  Port=3
  8 Engines : Gain  Gain=ones(1,8)  Multiplication=Matrix(K*u) (u vector)
  Mass : Gain  Gain=3491.05
  Ny wash : Subsystem
  Qbar Sref Cyb -1912 : Gain  Gain=-1912
  Slosh_Notch : Subsystem
  Sum : Sum  Inputs=-+|
  Sum2 : Sum  Inputs=-++
  Thrust : Gain  Gain=24890.1
  d2r : Gain  Gain=d2r
  betest : Outport
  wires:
  Sum/1 -> Mass/1
  r/1 -> Ny wash/1(in)
  Thrust/1 -> Sum2/2
  d2r/1 -> betest/1
  Mass/1 -> Sum2/1
  Ydd/1 -> Sum/2  "(ft/sec^2)"
  Qbar Sref Cyb -1912/1 -> Sum2/3
  Sum2/1 -> Slosh_Notch/1(in)  "(deg)"
  Ny wash/1(ou) -> Sum/1
  Slosh_Notch/1(ou) -> Qbar Sref Cyb -1912/1, d2r/1
  dz/1 -> 8 Engines/1  "(rad)"
  8 Engines/1 -> Thrust/1

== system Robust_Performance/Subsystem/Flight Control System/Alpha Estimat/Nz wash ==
  in : Inport
  3 : Gain  Gain=19
  Transfer Fcn : TransferFcn  Numerator="[1  0]"  Denominator="[0.015  1]"
  ou : Outport
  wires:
  in/1 -> Transfer Fcn/1
  Transfer Fcn/1 -> 3/1
  3/1 -> ou/1

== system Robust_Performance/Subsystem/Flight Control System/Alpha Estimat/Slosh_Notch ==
  in : Inport
  0.1 : Gain  Gain=0.00035
  Int1 : Integrator
  Transfer Fcn2 : TransferFcn  Numerator="[1 0.016*4.4  4.38^2]"  Denominator="[1  0.32*4.4  4.38^2]"
  ou : Outport
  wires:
  in/1 -> 0.1/1
  Transfer Fcn2/1 -> Int1/1
  0.1/1 -> Transfer Fcn2/1
  Int1/1 -> ou/1

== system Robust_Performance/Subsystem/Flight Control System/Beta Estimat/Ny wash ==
  in : Inport
  3 : Gain  Gain=19
  Transfer Fcn1 : TransferFcn  Numerator="[1  0]"  Denominator="[0.015  1]"
  ou : Outport
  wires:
  in/1 -> Transfer Fcn1/1
  Transfer Fcn1/1 -> 3/1
  3/1 -> ou/1

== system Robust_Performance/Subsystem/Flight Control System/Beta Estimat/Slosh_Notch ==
  in : Inport
  0.1 : Gain  Gain=0.00035
  Int1 : Integrator
  Transfer Fcn2 : TransferFcn  Numerator="[1 0.016*4.4  4.38^2]"  Denominator="[1  0.32*4.4  4.38^2]"
  ou : Outport
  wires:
  in/1 -> 0.1/1
  Int1/1 -> ou/1
  0.1/1 -> Transfer Fcn2/1
  Transfer Fcn2/1 -> Int1/1
